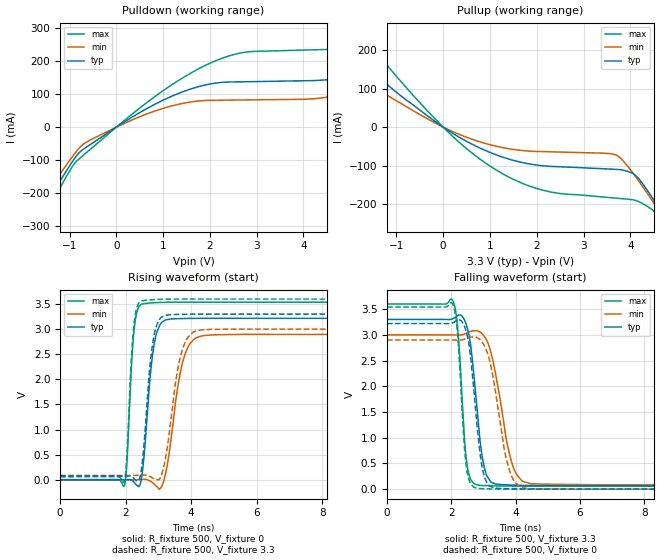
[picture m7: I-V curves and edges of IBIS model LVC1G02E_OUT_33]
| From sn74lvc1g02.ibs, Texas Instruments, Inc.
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[Model]   LVC1G02E_OUT_33
Model_type  Output
Vref =   0
Rref =   500
Cref =   50p
Vmeas =   1.5
| variable   typ   min   max
C_comp   7.76pF   3.46pF   12.81pF
| C_pullup   6.91pF   3.46pF   8.78pF
| C_pulldown   8.62pF   4.34pF   12.81pF
[Temperature Range]   40   100   -40
| Ambient temperature   25   85   -40
[Voltage range]   3.3   3   3.6
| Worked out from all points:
|   slope of the pulldown table from 0 to 0.495 V, typ, clamps not added: 11.3 ohm
|   slope of the pullup table from 0 to 0.495 V, typ, clamps not added: 13.5 ohm
|   rising waveform, R_fixture 500, V_fixture 0: 20-80 % time 256ps typ, 390ps min, 167ps max; typ from 0 V to 3.22 V
|   falling waveform, R_fixture 500, V_fixture 3.3: 20-80 % time 312ps typ, 495ps min, 208ps max; typ from 3.3 V to 0.069 V
|   rising waveform, R_fixture 500, V_fixture 3.3: 20-80 % time 251ps typ, 382ps min, 165ps max; typ from 0.069 V to 3.3 V
|   falling waveform, R_fixture 500, V_fixture 0: 20-80 % time 307ps typ, 460ps min, 205ps max; typ from 3.22 V to 0 V
[Pulldown]
| LVC1G02E_OUT_33
|   Voltage   I(typ)   I(min)   I(max)
-5.5V     -1.134A    -1.018A    -1.274A
-2.675V   -504.7mA   -448.2mA   -566.2mA
-1.54V    -241.1mA   -211.6mA   -271.3mA
-660mV    -62.57mA   -46.97mA   -79.82mA
1.92V     128.4mA    80.95mA    188.3mA
4.75V     148.7mA    96.8mA     237.9mA
6.03V     209.6mA    151.8mA    306.6mA
6.98V     278.7mA    201.6mA    396.3mA
7.35V     308.5mA    129.4mA    437mA
7.84V     330.1mA    92.52mA    494.2mA
8.75V     170.8mA    93.27mA    500.6mA
11V       160mA      96.49mA    276.8mA
[Pullup]
| LVC1G02E_OUT_33
|   Voltage   I(typ)   I(min)   I(max)
-5.5V     622.4mA    491.4mA    870.3mA
-3.265V   341.5mA    264.8mA    484.1mA
-2.52V    253.8mA    195mA      362.3mA
-1.98V    193mA      147.1mA    277.2mA
-175mV    14.9mA     10.92mA    21.78mA
1.005V    -65.77mA   -45.62mA   -101.2mA
2.125V    -100.1mA   -63.35mA   -163.2mA
3.695V    -109.4mA   -72.27mA   -184mA
4.115V    -125.2mA   -128.8mA   -190.1mA
4.73V     -232.9mA   -238mA     -260.1mA
4.9V      -266.3mA   -269.5mA   -295.7mA
11V       -1.559A    -1.467A    -1.714A
[Ramp]
| LVC1G02E_OUT_33
| variable   typ   min   max
dV/dt_r   2.01/2.69E-10   1.85/4.28E-10   2.20/1.74E-10
dV/dt_f   1.99/3.37E-10   1.80/5.46E-10   2.18/2.25E-10
R_load = 500
[Rising Waveform]
| LVC1G02E_OUT_33
R_fixture =   500
C_fixture =   0
L_fixture =   0
V_fixture =   0
V_fixture_min = 0
V_fixture_max = 0
|   Time   V(typ)   V(min)   V(max)
0s        141.8pV    4.978nV    2.659nV
1.965ns   371.1uV    -27.85uV   -112.3mV
2.035ns   1.293mV    -69.24uV   310.7mV
2.25ns    -45.05mV   -215uV     2.939V
2.515ns   181.4mV    4.744mV    3.503V
2.855ns   2.643V     -78.47mV   3.528V
3.25ns    3.191V     223.2mV    3.537V
3.755ns   3.213V     2.385V     3.54V
4.355ns   3.217V     2.871V     3.54V
24.99ns   3.216V     2.894V     3.539V
[Falling Waveform]
| LVC1G02E_OUT_33
R_fixture =   500
C_fixture =   0
L_fixture =   0
V_fixture =   3.3
V_fixture_min = 3
V_fixture_max = 3.6
|   Time   V(typ)   V(min)   V(max)
0s        3.3V       3V         3.6V
2.05ns    3.315V     2.998V     3.664V
2.205ns   3.378V     2.997V     3.087V
2.48ns    3.171V     3.036V     520.6mV
2.82ns    1.442V     3.075V     80.73mV
2.985ns   551.2mV    3.004V     70.04mV
3.2ns     166mV      2.729V     65.34mV
3.895ns   79.54mV    488.2mV    59.12mV
4.445ns   71.41mV    110.2mV    58.44mV
24.99ns   69.39mV    85.92mV    58.95mV
[Rising Waveform]
| LVC1G02E_OUT_33
R_fixture =   500
C_fixture =   0
L_fixture =   0
V_fixture =   3.3
V_fixture_min = 3
V_fixture_max = 3.6
|   Time   V(typ)   V(min)   V(max)
0s        69.35mV    85.87mV    58.92mV
1.955ns   69.65mV    85.85mV    -42.1mV
2.03ns    70.45mV    85.81mV    409.8mV
2.24ns    34.56mV    85.64mV    3.012V
2.49ns    257.3mV    89.4mV     3.565V
2.83ns    2.743V     30.85mV    3.589V
3.225ns   3.28V      463.6mV    3.598V
3.7ns     3.296V     2.527V     3.601V
4.28ns    3.301V     2.985V     3.601V
24.99ns   3.3V       3V         3.6V
[Falling Waveform]
| LVC1G02E_OUT_33
R_fixture =   500
C_fixture =   0
L_fixture =   0
V_fixture =   0
V_fixture_min = 0
V_fixture_max = 0
|   Time   V(typ)   V(min)   V(max)
0s        3.22V      2.9V       3.542V
2.045ns   3.233V     2.899V     3.595V
2.19ns    3.284V     2.897V     3.055V
2.47ns    3.047V     2.93V      425.1mV
2.81ns    1.179V     2.943V     17.24mV
2.955ns   443.4mV    2.863V     9.233mV
3.125ns   110.5mV    2.648V     6.161mV
3.75ns    7.995mV    493.9mV    683.5uV
4.23ns    2.488mV    23.27mV    -217.8uV
24.99ns   35.15uV    43.43uV    31.92uV
